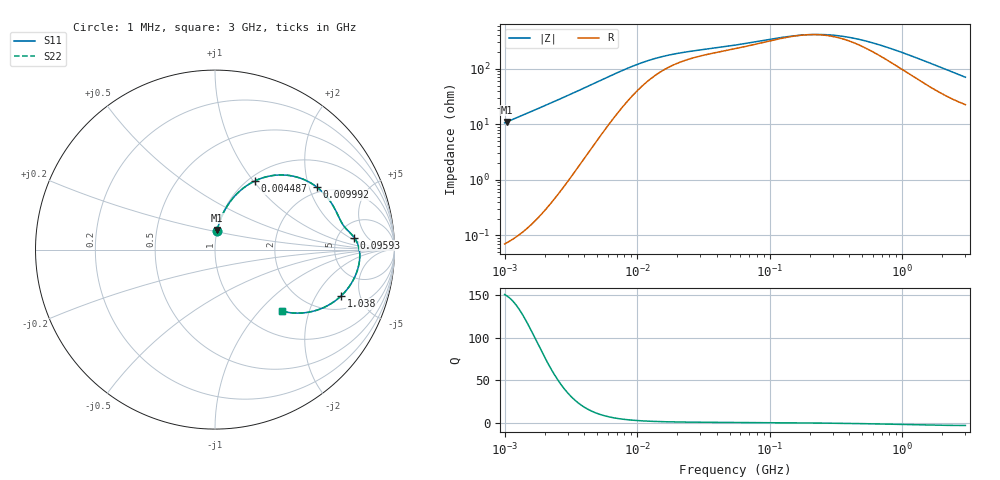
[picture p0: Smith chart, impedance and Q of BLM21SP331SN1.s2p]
! BLM21SP331SN1
# Hz S RI R 50
!Freq.(Hz) S11(Real) S11(Imag) S21(Real) S21(Imag) S12(Real) S12(Imag) S22(Real) S22(Imag)
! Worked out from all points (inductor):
!   401 points, 1 MHz to 3 GHz, reference 50 ohm
!   read as one part in series: L = 1.7 uH near 1.041 MHz
!   highest Q = 149 at 1.041 MHz (marker M1), where L = 1.69 uH
!   self-resonance near 193.2 MHz
!   S11 on the Smith chart (normalised r, x): 1 MHz: 1.00, +0.21; 4.487 MHz: 1.07, +1.02; 9.992 MHz: 1.80, +2.25; 95.93 MHz: 7.19, +2.44; 1.038 GHz: 2.83, -3.32; 3 GHz: 1.45, -1.33
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1000000  0.0119 0.105  0.9881 -0.105  0.9881 -0.105  0.0119 0.105
1040844  0.0128 0.1092  0.9872 -0.1092  0.9872 -0.1092  0.0128 0.1092
2271982  0.0606 0.2307  0.9394 -0.2307  0.9394 -0.2307  0.0606 0.2307
3006797  0.106 0.2938  0.894 -0.2938  0.894 -0.2938  0.106 0.2938
3823119  0.1682 0.3504  0.8318 -0.3504  0.8318 -0.3504  0.1682 0.3504
4487043  0.2245 0.3835  0.7755 -0.3835  0.7755 -0.3835  0.2245 0.3835
5481359  0.3103 0.4109  0.6897 -0.4109  0.6897 -0.4109  0.3103 0.4109
6563319  0.3954 0.4149  0.6046 -0.4149  0.6046 -0.4149  0.3954 0.4149
9992459  0.5665 0.3489  0.4335 -0.3489  0.4335 -0.3489  0.5665 0.3489
1.461624e7  0.6487 0.2589  0.3513 -0.2589  0.3513 -0.2589  0.6487 0.2589
2.559965e7  0.697 0.1667  0.303 -0.1667  0.303 -0.1667  0.697 0.1667
5.477226e7  0.74 0.1061  0.26 -0.1061  0.26 -0.1061  0.74 0.1061
9.593103e7  0.7757 0.067  0.2243 -0.067  0.2243 -0.067  0.7757 0.067
1.49005e8  0.7968 0.027  0.2032 -0.027  0.2032 -0.027  0.7968 0.027
2.094008e8  0.8052 -0.00886  0.1948 0.00886  0.1948 0.00886  0.8052 -0.00886
2.827291e8  0.8065 -0.0442  0.1935 0.0442  0.1935 0.0442  0.8065 -0.0442
3.894533e8  0.8009 -0.0868  0.1991 0.0868  0.1991 0.0868  0.8009 -0.0868
5.364635e8  0.7858 -0.1362  0.2142 0.1362  0.2142 0.1362  0.7858 -0.1362
8.005644e8  0.7461 -0.2083  0.2539 0.2083  0.2539 0.2083  0.7461 -0.2083
1.038491e9  0.7021 -0.2584  0.2979 0.2584  0.2979 0.2584  0.7021 -0.2584
1.855641e9  0.54 -0.3449  0.46 0.3449  0.46 0.3449  0.54 -0.3449
3e9  0.3708 -0.3425  0.6292 0.3425  0.6292 0.3425  0.3708 -0.3425
